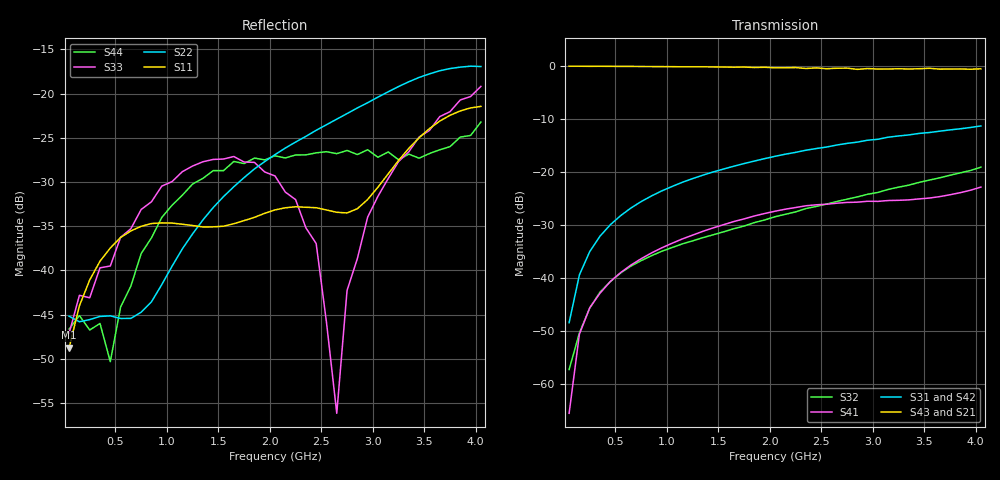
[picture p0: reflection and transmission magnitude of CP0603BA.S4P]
! Network Analyzer HP8720D.07.14 Serial No. US38111185
! 28 Apr 1999  02:06:29
! Frequency 	S11		S21		S31		S41		S12		S22		S23		S24		S13		S23		S33		S34		S14		S24		S34		S44
# HZ  S  DB R 50
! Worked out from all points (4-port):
!   41 points, 50 MHz to 4.05 GHz, reference 50 ohm
!   strongest paths, dB at 50 MHz, 1.05 GHz, 2.05 GHz, 3.05 GHz, 4.05 GHz:
!     S43: 0.0, -0.1, -0.3, -0.5, -0.5
!     S21: 0.0, -0.1, -0.3, -0.6, -0.8
!     S31: -48.3, -22.7, -17.0, -13.8, -11.3
!     S42: -47.0, -22.7, -17.0, -13.7, -11.3
!     S41: -65.4, -33.4, -27.3, -25.5, -22.8
!     S32: -57.2, -34.2, -28.4, -23.8, -19.0
!   lowest |S11| = -48.7 dB at 50 MHz (marker M1), VSWR 1.01, Z = 50.4 - j0.0205 ohm
!   |S11| at or under -10 dB: start of sweep to end of sweep
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5e7  -48.75 -3.2  0.01 -1.0  -50.21 89.3  -60.66 115.0
     0.01 -0.7  -45.17 5.1  -54.52 82.1  -47.96 93.8
     -48.34 87.2  -57.19 131.2  -47.10 1.7  -0.00 -1.1
     -65.45 104.8  -47.03 100.3  0.02 -0.8  -46.64 -1.6
4.5e8  -37.46 -85.4  -0.02 -6.4  -29.93 82.8  -40.63 83.6
       -0.01 -6.6  -45.13 -23.9  -40.66 80.6  -29.98 82.8
       -29.89 82.5  -40.61 80.6  -39.50 73.4  -0.02 -7.0
       -40.59 83.5  -29.99 82.7  -0.01 -7.1  -50.32 73.0
1.85e9  -34.00 -103.0  -0.21 -25.9  -17.83 62.4  -28.21 64.0
        -0.27 -26.6  -28.53 -9.3  -29.58 70.8  -17.93 62.8
        -17.87 62.3  -29.47 71.3  -27.78 87.4  -0.19 -28.1
        -28.23 64.3  -17.88 62.3  -0.23 -28.8  -27.30 132.4
2.45e9  -32.91 -88.8  -0.39 -34.2  -15.48 53.7  -26.11 51.8
        -0.37 -35.0  -24.16 -27.2  -26.52 67.0  -15.65 54.4
        -15.51 53.1  -26.44 66.7  -36.96 89.4  -0.39 -37.3
        -26.12 51.4  -15.52 53.1  -0.30 -37.6  -26.71 155.4
2.65e9  -33.43 -75.5  -0.40 -36.9  -14.84 50.4  -25.78 48.3
        -0.45 -37.4  -22.90 -29.1  -25.56 64.7  -15.02 51.2
        -14.85 50.5  -25.49 64.9  -56.15 70.4  -0.39 -40.2
        -25.82 48.2  -14.87 50.3  -0.37 -40.3  -26.80 163.8
2.95e9  -31.98 -39.4  -0.50 -41.3  -14.00 45.8  -25.43 44.5
        -0.50 -41.1  -21.04 -30.0  -24.24 61.5  -14.21 46.7
        -13.94 46.2  -24.13 61.9  -33.97 -97.1  -0.49 -44.7
        -25.45 44.5  -13.98 46.0  -0.42 -44.2  -26.35 177.4
4.05e9  -21.45 -10.4  -1.19 -59.7  -11.65 28.3  -22.76 46.7
        -0.76 -54.7  -16.95 -39.3  -19.26 42.6  -11.90 30.8
        -11.25 32.2  -19.02 45.9  -19.20 -102.3  -1.11 -64.2
        -22.78 48.6  -11.30 32.3  -0.47 -58.5  -23.23 -134.9
